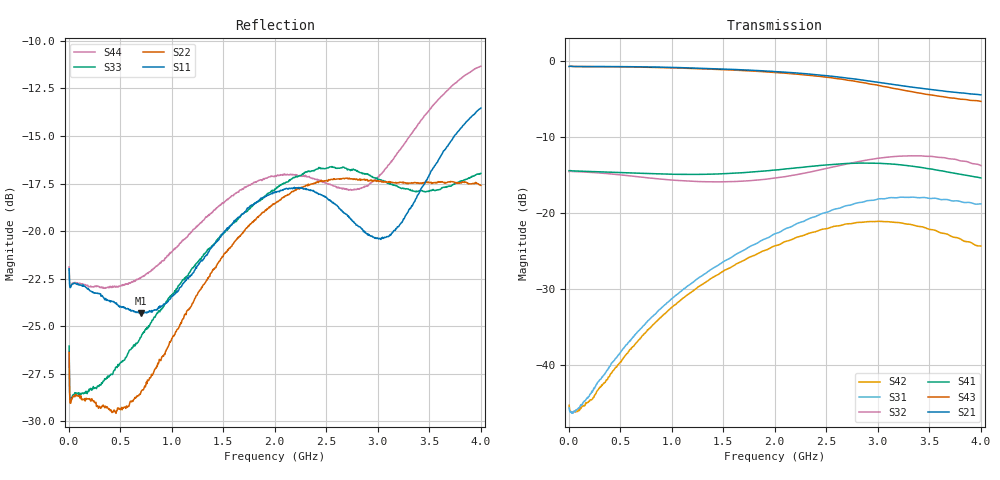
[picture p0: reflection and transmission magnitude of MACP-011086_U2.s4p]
!Agilent Technologies,E5071C,MY46110647,A.11.31
!Date: Thu Jul 09 12:04:52 2020 DD
!Data & Calibration Information:
!MACP-011086 soldered onto PT-0010289 with SMA connectors, calibration PCB PT-0003654. Port1 (pin1) Port2 (pin5) Port3 (pin4) Port4 (pin3)
!Freq	S11:SOLT4(ON)	S12:SOLT4(ON)	S13:SOLT4(ON)	S14:SOLT4(ON)
!	S21:SOLT4(ON)	S22:SOLT4(ON)	S23:SOLT4(ON)	S24:SOLT4(ON)
!	S31:SOLT4(ON)	S32:SOLT4(ON)	S33:SOLT4(ON)	S34:SOLT4(ON)
!	S41:SOLT4(ON)	S42:SOLT4(ON)	S43:SOLT4(ON)	S44:SOLT4(ON)
!PortZ  Port1:50+j0  Port2:50+j0  Port3:50+j0  Port4:50+j0
!Above PortZ is port z conversion or system Z0 setting when saving the data.
!When reading, reference impedance value at option line is always used.
# Hz S MA R 50
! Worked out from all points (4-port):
!   800 points, 5 MHz to 4 GHz, reference 50 ohm
!   strongest paths, dB at 5 MHz, 1.005 GHz, 2.005 GHz, 3.005 GHz, 4 GHz:
!     S21: -0.7, -0.8, -1.4, -2.8, -4.4
!     S43: -0.7, -0.9, -1.5, -3.2, -5.3
!     S41: -14.4, -14.9, -14.3, -13.4, -15.4
!     S32: -14.6, -15.7, -15.4, -12.8, -13.8
!     S31: -45.7, -31.3, -22.7, -18.2, -18.8
!     S42: -45.4, -32.4, -24.3, -21.1, -24.4
!   lowest |S11| = -24.3 dB at 705 MHz (marker M1), VSWR 1.13, Z = 48.9 + j5.93 ohm
!   |S11| at or under -10 dB: start of sweep to end of sweep
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5000000  0.07973 158.3  0.9258 1.6  0.00453 179.3  0.1893 -178.8
         0.9252 1.6  0.04801 140.8  0.1873 1.8  0.004669 170.9
         0.005179 178.9  0.187 1.8  0.04989 141.2  0.924 1.6
         0.1899 -178.7  0.00538 177.6  0.9237 1.6  0.08061 158.0
2.25e8  0.06926 154.9  0.923 -5.9  0.006298 -169.8  0.1871 164.9
        0.9231 -5.9  0.03628 146.6  0.1852 -4.8  0.005699 179.6
        0.006675 -171.6  0.1849 -4.8  0.0382 140.7  0.9212 -6.0
        0.1874 164.9  0.005869 176.9  0.9215 -6.0  0.07142 151.0
7.05e8  0.06079 96.7  0.9192 -18.7  0.01698 159.4  0.1826 134.5
        0.9188 -18.7  0.03798 71.4  0.1724 -12.2  0.01496 147.1
        0.01735 158.4  0.1723 -12.1  0.05281 76.2  0.9149 -18.9
        0.1825 134.5  0.01513 147.4  0.9144 -18.9  0.07572 90.8
1.415e9  0.09249 14.8  0.8942 -38.0  0.04283 107.1  0.1809 94.1
         0.8935 -38.0  0.0796 6.7  0.1602 -15.4  0.03768 98.3
         0.04376 107.4  0.1604 -15.2  0.09291 19.1  0.8857 -38.3
         0.1805 94.2  0.03807 98.5  0.8854 -38.3  0.1136 24.3
2.46e9  0.1241 -35.7  0.8096 -67.2  0.09949 34.7  0.2069 32.3
        0.8088 -67.2  0.1353 -31.1  0.1931 -20.0  0.07727 30.1
        0.09921 35.9  0.1936 -20.2  0.1461 -34.2  0.7935 -68.1
        0.2062 32.8  0.07798 30.6  0.791 -68.1  0.1352 -12.3
3.11e9  0.0973 -19.5  0.7106 -84.2  0.1291 -21.6  0.2114 -17.2
        0.7094 -84.3  0.1351 -45.1  0.2342 -38.4  0.08722 -23.1
        0.1258 -19.7  0.2339 -38.7  0.1337 -55.0  0.6755 -85.6
        0.2107 -16.5  0.08741 -22.4  0.6724 -85.5  0.1497 4.9
4e9  0.2107 -17.2  0.6065 -102.8  0.1205 -108.7  0.1712 -90.7
     0.6002 -102.9  0.132 -69.7  0.2062 -79.3  0.0622 -112.4
     0.1145 -107.6  0.2052 -79.8  0.1419 -58.1  0.5478 -101.3
     0.1701 -89.7  0.06043 -111.9  0.5438 -100.8  0.2714 -6.6
